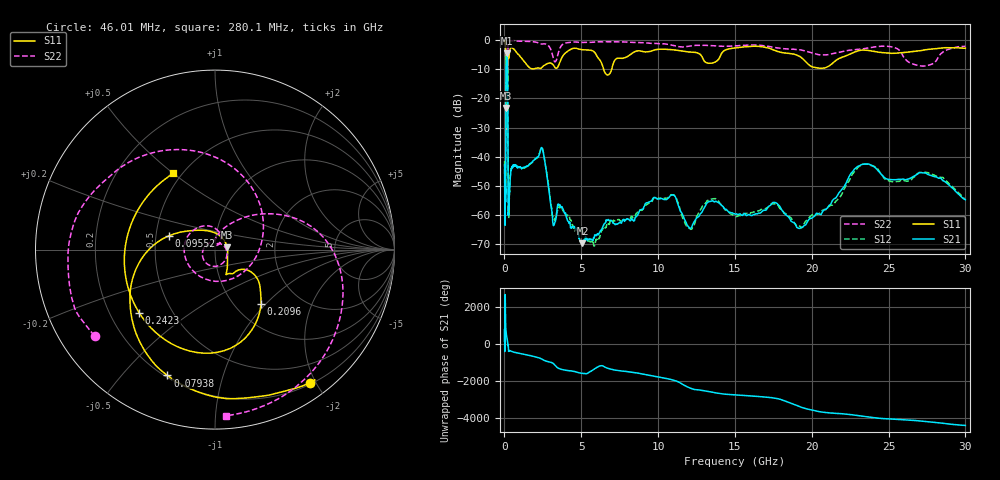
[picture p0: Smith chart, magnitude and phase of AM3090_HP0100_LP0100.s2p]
! Date/Time: Thu, Feb 28, 2019 1:57 PM
! Network Analyzer: Agilent Technologies E8364B Rev: A.07.50.67
! Sweep from 0.010 to 30.000 GHz, 1601 Points, Sweep Type: LOG
! Power Supply: 5.023 V, 0.002 A
# Hz S DB R 50
!freq MagS11 AngS11 MagS21 AngS21 MagS12 AngS12 MagS22 AngS22
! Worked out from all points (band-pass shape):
!   1601 points, 10 MHz to 30 GHz, reference 50 ohm
!   highest |S21| = -4.54 dB at 145.4 MHz (marker M1); lowest = -69.7 dB at 5.077 GHz (marker M2)
!   |S21| within 3 dB of the highest: 105.1 MHz to 196.9 MHz (91.78 MHz wide, 60.8 % of centre)
!   lowest |S11| = -23.3 dB at 103.5 MHz (marker M3), VSWR 1.15, Z = 57.2 + j1.53 ohm
!   |S11| at or under -10 dB: 94.63 MHz to 200.2 MHz (105.5 MHz wide, 71.6 % of centre); 6.455 GHz to 6.977 GHz (521.3 MHz wide, 7.76 % of centre)
!   |S22| runs from -32.6 to -0.1 dB; largest |S21 - S12| = 0.014
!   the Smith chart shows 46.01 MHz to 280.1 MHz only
!   S11 on the Smith chart (normalised r, x): 46.01 MHz: 0.21, -1.92; 79.38 MHz: 0.21, -0.67; 95.52 MHz: 0.59, +0.10; 209.6 MHz: 1.31, -0.93; 242.3 MHz: 0.32, -0.33; 280.1 MHz: 0.45, +0.50
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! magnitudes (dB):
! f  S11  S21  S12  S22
! 10 MHz  -0.3  -42.7  -41.5  -0.5
! 38.04 MHz  -0.5  -62.0  -60.8  -1.3
! 46.01 MHz  -0.8  -51.2  -52.3  -1.7
! 79.38 MHz  -2.5  -48.3  -48.3  -5.0
! 95.52 MHz  -11.4  -15.4  -15.3  -15.2
! 103.5 MHz  -23.3  -8.2  -8.2  -15.6
! 129 MHz  -16.3  -4.8  -4.8  -32.4
! 144.7 MHz  -16.1  -4.5  -4.5  -24.6
! 145.4 MHz  -16.1  -4.5  -4.5  -24.3
! 186.8 MHz  -13.9  -6.0  -6.0  -26.4
! 209.6 MHz  -8.1  -13.0  -13.0  -11.6
! 242.3 MHz  -5.2  -55.4  -54.1  -1.5
! 280.1 MHz  -6.3  -57.8  -60.7  -0.7
! 550.5 MHz  -2.9  -43.4  -43.1  -0.2
! 2.084 GHz  -9.7  -40.4  -40.5  -0.8
! 2.47 GHz  -9.3  -37.3  -37.1  -1.4
! 3.204 GHz  -8.7  -63.5  -61.3  -6.7
! 5.077 GHz  -3.3  -69.7  -65.4  -0.8
! 7.926 GHz  -5.9  -61.5  -61.5  -0.7
! 19.41 GHz  -6.4  -64.2  -63.8  -3.5
! 23.48 GHz  -3.5  -42.6  -42.5  -2.9
! 30 GHz  -2.8  -54.8  -54.7  -2.2
